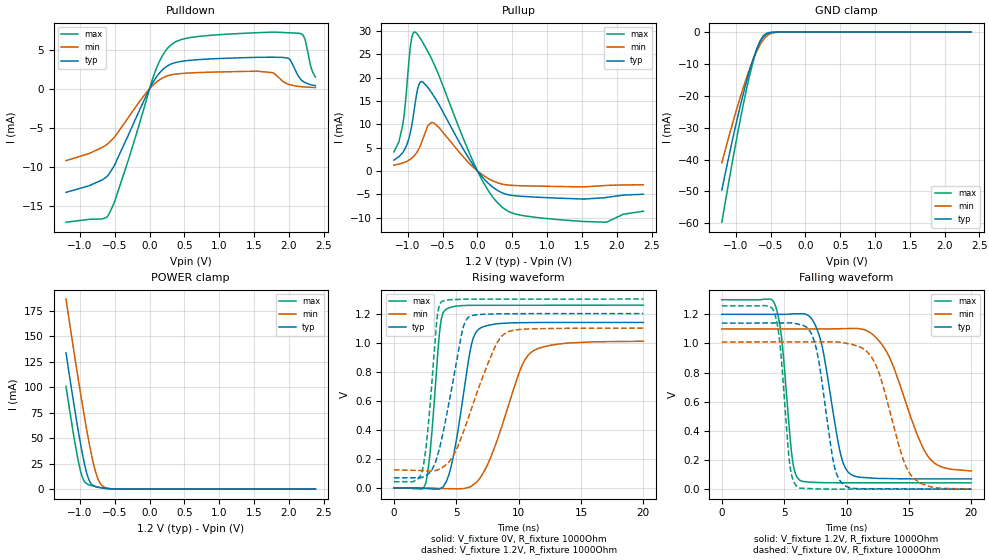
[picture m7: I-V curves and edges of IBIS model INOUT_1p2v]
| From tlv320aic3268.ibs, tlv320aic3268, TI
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|   INOUT_1p2v
[Model]   INOUT_1p2v
Model_type   I/O
Polarity   Non-Inverting
Enable   Active-High
Vinl = 0.12
Vinh = 1.08
Vmeas = 0.6
Vref = 0
Cref = 5pF
Rref = 10000
|   typ   min   max
C_comp   1.460pF   1.439pF   1.501pF
[Voltage Range]   1.2   1.1   1.3
[Temperature Range]   27   125   -40
[Pullup Reference]   1.2   1.1   1.3
[Pulldown Reference]   -0   -0   -0
[Power Clamp Reference]   1.2   1.1   1.3
[GND Clamp Reference]   -0   -0   -0
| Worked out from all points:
|   slope of the pulldown table from 0 to 0.18 V, typ, clamps not added: 75.7 ohm
|   slope of the pullup table from 0 to 0.18 V, typ, clamps not added: 60.4 ohm
|   GND clamp passes 1 mA (typ) near -0.58 V on its own axis
|   POWER clamp passes 1 mA (typ) near -0.66 V on its own axis
|   falling waveform, V_fixture 1.2V, R_fixture 1000Ohm: 20-80 % time 1.33ns typ, 2.49ns min, 761ps max; typ from 1.2 V to 0.07 V
|   rising waveform, V_fixture 0V, R_fixture 1000Ohm: 20-80 % time 1.26ns typ, 2.38ns min, 684ps max; typ from 0 V to 1.14 V
|   rising waveform, V_fixture 1.2V, R_fixture 1000Ohm: 20-80 % time 1.52ns typ, 2.5ns min, 741ps max; typ from 0.07 V to 1.2 V
|   falling waveform, V_fixture 0V, R_fixture 1000Ohm: 20-80 % time 1.16ns typ, 1.98ns min, 703ps max; typ from 1.14 V to 0 V
[Pulldown]
|   Voltage   I(typ)   I(min)   I(max)
-1.2V     -13.2mA    -9.162mA   -17.01mA
-588mV    -10.94mA   -6.92mA    -16.07mA
-300mV    -5.802mA   -3.6mA     -8.956mA
96mV      1.476mA    836.3uA    2.556mA
366mV     3.329mA    1.866mA    5.948mA
1.554V    4.018mA    2.238mA    7.16mA
1.914V    4.005mA    932.7uA    7.184mA
2.022V    3.684mA    492.9uA    7.135mA
2.166V    1.251mA    281.4uA    7.05mA
2.22V     853.1uA    240.5uA    6.591mA
2.31V     534.9uA    192.7uA    3.013mA
2.382V    406.2uA    165.9uA    1.498mA
[GND Clamp]
|   Voltage   I(typ)   I(min)   I(max)
-1.2V     -49.54mA   -41.02mA   -59.63mA
-1.11V    -40.13mA   -33.68mA   -48.23mA
-984mV    -27.71mA   -23.98mA   -33.03mA
-894mV    -19.56mA   -17.57mA   -22.98mA
-822mV    -13.63mA   -12.87mA   -15.63mA
-750mV    -8.449mA   -8.649mA   -9.209mA
-696mV    -5.221mA   -5.912mA   -5.279mA
-642mV    -2.747mA   -3.65mA    -2.42mA
-588mV    -1.156mA   -1.964mA   -813.9uA
-498mV    -158.5uA   -480.1uA   -66.74uA
-390mV    -7.515uA   -52.8uA    -1.231uA
2.382V    0A         0A         0A
[Pullup]
|   Voltage   I(typ)   I(min)   I(max)
-1.2V     2.325mA    1.228mA    4.085mA
-1.074V   3.929mA    1.705mA    9.791mA
-966mV    8.071mA    2.5mA      26.37mA
-930mV    10.96mA    2.931mA    29.35mA
-894mV    14.6mA     3.508mA    29.77mA
-858mV    17.67mA    4.294mA    29.24mA
-804mV    19.17mA    6.03mA     28.01mA
-642mV    16.4mA     10.36mA    23.49mA
6mV       -118.8uA   -73.78uA   -185.7uA
366mV     -4.756mA   -2.854mA   -7.904mA
1.842V    -5.72mA    -3.115mA   -10.99mA
2.382V    -4.999mA   -2.958mA   -8.643mA
[POWER Clamp]
|   Voltage   I(typ)   I(min)   I(max)
-1.2V     133.6mA    186.3mA    100.7mA
-1.056V   70.3mA     121.7mA    39.38mA
-1.002V   48.47mA    98.42mA    20.74mA
-966mV    35.1mA     83.35mA    11.87mA
-912mV    18.12mA    61.68mA    5.82mA
-858mV    7.384mA    41.68mA    4.055mA
-804mV    3.295mA    24.42mA    3.025mA
-768mV    2.316mA    15.25mA    2.436mA
-732mV    1.752mA    8.564mA    1.901mA
-678mV    1.158mA    3.201mA    1.207mA
-444mV    33.19uA    98.2uA     12.33uA
2.382V    0A         0A         0A
[Ramp]
R_load = 1000
|   typ   min   max
dV/dt_r   0.683621/1.2582e-009   0.604954/2.384e-009   0.754869/6.83404e-010
dV/dt_f   0.677797/1.32597e-009  0.585074/2.48199e-009  0.754006/7.58939e-010
[Falling Waveform]
V_fixture = 1.2V
V_fixture_min = 1.1V
V_fixture_max = 1.3V
R_fixture = 1000Ohm
C_fixture = 0F
|   Time   V(typ)   V(min)   V(max)
0s        1.2V       1.1V       1.3V
4.259ns   1.2V       1.1V       1.267V
4.805ns   1.2V       1.1V       1.029V
5.678ns   1.203V     1.1V       191.9mV
6.259ns   1.204V     1.1V       60.78mV
7.789ns   1.061V     1.1V       45.48mV
10.09ns   121.2mV    1.102V     43.97mV
13.15ns   72.9mV     952.7mV    43.77mV
16.61ns   70.62mV    215.9mV    43.54mV
20ns      70.34mV    124.8mV    43.32mV
[Rising Waveform]
V_fixture = 0V
V_fixture_min = 0V
V_fixture_max = 0V
R_fixture = 1000Ohm
C_fixture = 0F
|   Time   V(typ)   V(min)   V(max)
0s        -83.19nV   1.471mV    238.7nV
2.541ns   -3.499mV   755.8uV    31.31mV
2.98ns    -5.929mV   -341.9uV   319.8mV
3.723ns   -3.176mV   -3.412mV   1.12V
4.182ns   43.4mV     -4.177mV   1.23V
4.831ns   245.8mV    -5.256mV   1.249V
6.231ns   992.1mV    14.2mV     1.257V
6.775ns   1.091V     55.11mV    1.257V
10.99ns   1.138V     932.4mV    1.257V
20ns      1.139V     1.01V      1.258V
[Rising Waveform]
V_fixture = 1.2V
V_fixture_min = 1.1V
V_fixture_max = 1.3V
R_fixture = 1000Ohm
C_fixture = 0F
|   Time   V(typ)   V(min)   V(max)
0s        70.34mV    125.1mV    43.32mV
2.251ns   72.84mV    119.8mV    111.9mV
2.7ns     93.47mV    117.9mV    382.2mV
3.475ns   217.1mV    124mV      1.177V
3.876ns   356.1mV    140.5mV    1.285V
5.496ns   1.085V     368.8mV    1.298V
6.095ns   1.182V     514.9mV    1.299V
8.034ns   1.198V     957.2mV    1.299V
9.061ns   1.199V     1.072V     1.299V
20ns      1.2V       1.1V       1.3V
[Falling Waveform]
|Gnd
V_fixture = 0V
V_fixture_min = 0V
V_fixture_max = 0V
R_fixture = 1000Ohm
C_fixture = 0F
|   Time   V(typ)   V(min)   V(max)
0s        1.139V     1.01V      1.258V
4.182ns   1.14V      1.01V      1.218V
4.681ns   1.141V     1.01V      979.1mV
5.433ns   1.141V     1.01V      180.4mV
6.112ns   1.133V     1.011V     12.8mV
7.505ns   988mV      1.011V     2.454mV
9.597ns   44.78mV    1.007V     529.4uV
12.29ns   2.673mV    863mV      392.5uV
15.18ns   1.671mV    94.03mV    245.4uV
20ns      -99.36nV   1.428mV    164.2nV
